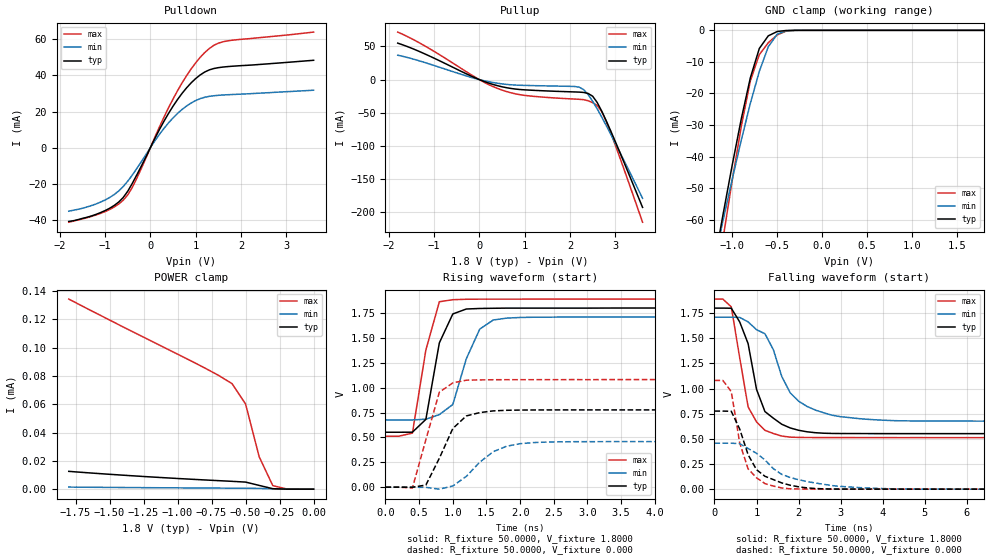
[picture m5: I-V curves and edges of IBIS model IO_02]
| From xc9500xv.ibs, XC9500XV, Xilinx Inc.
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|   Model IO_02
[Model]   IO_02
Model_type   I/O
Polarity   Non-Inverting
Enable   Active-High
Vinl =   0.8000V
Vinh =   2.0000V
Vmeas =   0.9000V
Cref =  35.0000pF
Rref =   1.0000M
Vref =  0.000V
C_comp   1.8820pF   1.2910pF   2.4730pF
[Temperature Range]   25.0000   100.0000   0.000
[Voltage Range]   1.8000V   1.7100V   1.8900V
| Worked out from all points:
|   slope of the pulldown table from 0 to 0.27 V, typ, clamps not added: 20.4 ohm
|   slope of the pullup table from 0 to 0.27 V, typ, clamps not added: 40.8 ohm
|   GND clamp passes 1 mA (typ) near -0.55 V on its own axis
|   rising waveform, R_fixture 50.0000, V_fixture 1.8000: 20-80 % time 238ps typ, 321ps min, 239ps max; typ from 0.552 V to 1.8 V
|   rising waveform, R_fixture 50.0000, V_fixture 0.000: 20-80 % time 351ps typ, 468ps min, 270ps max; typ from 0 V to 0.776 V
|   falling waveform, R_fixture 50.0000, V_fixture 1.8000: 20-80 % time 468ps typ, 728ps min, 362ps max; typ from 1.8 V to 0.552 V
|   falling waveform, R_fixture 50.0000, V_fixture 0.000: 20-80 % time 543ps typ, 1.06ns min, 348ps max; typ from 0.776 V to 0 V
[Pulldown]
| voltage   I(typ)   I(min)   I(max)
-1.8V     -40.9mA    -35.2mA    -41.3mA
-1.3V     -37.85mA   -32.1mA    -38.1mA
-900mV    -33.61mA   -27.65mA   -34.3mA
-700mV    -30.16mA   -24.04mA   -31.27mA
-500mV    -24.2mA    -18.6mA    -26.23mA
-300mV    -15.14mA   -11.58mA   -16.99mA
200mV     10.04mA    7.385mA    11.51mA
500mV     22.99mA    16.49mA    26.96mA
900mV     35.93mA    24.75mA    43.66mA
1.3V      43.1mA     28.44mA    54.96mA
1.7V      44.91mA    29.32mA    59.17mA
3.6V      48.42mA    31.83mA    64.04mA
[Pullup]
| voltage   I(typ)   I(min)   I(max)
-1.8V     54.98mA    36.8mA     71.63mA
-1.2V     38.67mA    25.69mA    50.7mA
-100mV    2.906mA    1.804mA    4.051mA
400mV     -9.157mA   -5.475mA   -13.28mA
1V        -15.43mA   -8.73mA    -23.81mA
2.2V      -18.82mA   -11.34mA   -29.66mA
2.4V      -20.89mA   -22.62mA   -31.86mA
2.5V      -25.06mA   -32.71mA   -34.73mA
2.6V      -34.53mA   -44.2mA    -38.98mA
2.7V      -47.58mA   -56.51mA   -48.25mA
2.9V      -77.68mA   -82.5mA    -80.44mA
3.6V      -192.6mA   -178.9mA   -214.9mA
[GND_clamp]
| voltage   I(typ)   I(min)   I(max)
-1.8V     -171.6mA   -154.7mA   -199.4mA
-1.2V     -73.41mA   -72.77mA   -83.79mA
-1.1V     -57.66mA   -59.67mA   -65.18mA
-1V       -42.38mA   -46.9mA    -47.16mA
-900mV    -27.9mA    -34.63mA   -30.27mA
-800mV    -15.03mA   -23.14mA   -16.01mA
-700mV    -5.733mA   -12.98mA   -7.683mA
-600mV    -1.741mA   -5.183mA   -3.919mA
-500mV    -371uA     -1.195mA   -1.434mA
-400mV    -43.13uA   -156.2uA   -255.7uA
-200mV    -89.07nA   -475.8nA   -857.8nA
1.8V      335.2pA    7.048nA    1.584nA
[POWER_clamp]
| voltage   I(typ)   I(min)   I(max)
-1.8V     12.57uA    1.465uA    134.2uA
-800mV    6.509uA    806.2nA    85.56uA
-600mV    5.531uA    702nA      74.53uA
-500mV    4.994uA    650.2nA    60.11uA
-400mV    2.651uA    538.7nA    22.85uA
-300mV    324.7nA    232.1nA    2.491uA
-200mV    23.09nA    31.76nA    201.3nA
0V        335.2pA    3.931nA    2.177nA
[Ramp]
| variable   typ   min   max
dV/dt_r   0.4658/0.2913n   0.2744/0.4008n   0.6486/0.2153n
dV/dt_f   0.7489/0.4235n   0.6203/0.6773n   0.8266/0.3232n
R_load = 50.0000
[Rising Waveform]
R_fixture = 50.0000
V_fixture = 1.8000
V_fixture_min = 1.7100
V_fixture_max = 1.8900
L_fixture = 0.000H
C_fixture = 0.000F
| time   V(typ)   V(min)   V(max)
0s        551.9mV    676mV      512.4mV
400ps     552.6mV    675.8mV    543.2mV
600ps     681.4mV    683.2mV    1.379V
800ps     1.45V      729.3mV    1.863V
1ns       1.74V      830.8mV    1.884V
1.2ns     1.79V      1.289V     1.888V
1.4ns     1.796V     1.588V     1.889V
1.6ns     1.798V     1.679V     1.889V
2.6ns     1.799V     1.709V     1.89V
10ns      1.8V       1.71V      1.89V
[Rising Waveform]
R_fixture = 50.0000
V_fixture = 0.000
V_fixture_min = 0.000
V_fixture_max = 0.000
L_fixture = 0.000H
C_fixture = 0.000F
| time   V(typ)   V(min)   V(max)
0s        0V         0V         0V
400ps     -693.6uV   8.399uV    -8.012mV
600ps     21.47mV    -1.641mV   477.8mV
800ps     290.8mV    -19.95mV   954mV
1ns       589.4mV    12.4mV     1.048V
1.2ns     715.8mV    107.8mV    1.075V
1.6ns     766.5mV    356.6mV    1.079V
1.8ns     772.5mV    411.6mV    1.08V
2.2ns     775.7mV    448.3mV    1.08V
10ns      776.3mV    457.4mV    1.081V
[Falling Waveform]
R_fixture = 50.0000
V_fixture = 1.8000
V_fixture_min = 1.7100
V_fixture_max = 1.8900
L_fixture = 0.000H
C_fixture = 0.000F
| time   V(typ)   V(min)   V(max)
0s        1.8V       1.71V      1.89V
400ps     1.799V     1.71V      1.812V
600ps     1.663V     1.708V     1.307V
800ps     1.447V     1.663V     817.9mV
1ns       992.3mV    1.586V     669mV
1.2ns     771.4mV    1.545V     585.1mV
1.4ns     705.6mV    1.387V     553.4mV
1.8ns     608.8mV    958.2mV    517.3mV
2.8ns     554mV      734.9mV    512.9mV
10ns      551.9mV    676.2mV    512.4mV
[Falling Waveform]
R_fixture = 50.0000
V_fixture = 0.000
V_fixture_min = 0.000
V_fixture_max = 0.000
L_fixture = 0.000H
C_fixture = 0.000F
| time   V(typ)   V(min)   V(max)
0s        776.3mV    457mV      1.081V
200ps     776.3mV    457mV      1.081V
400ps     774.2mV    457mV      969.4mV
600ps     598.1mV    452.3mV    460.4mV
800ps     342.4mV    404.2mV    201.5mV
1ns       193.4mV    357mV      113.3mV
1.4ns     95.11mV    203.6mV    30.94mV
2ns       23.37mV    93.99mV    1.795mV
3.4ns     698.1uV    16.74mV    139.5uV
10ns      30.33uV    124.3uV    -2.557uV
